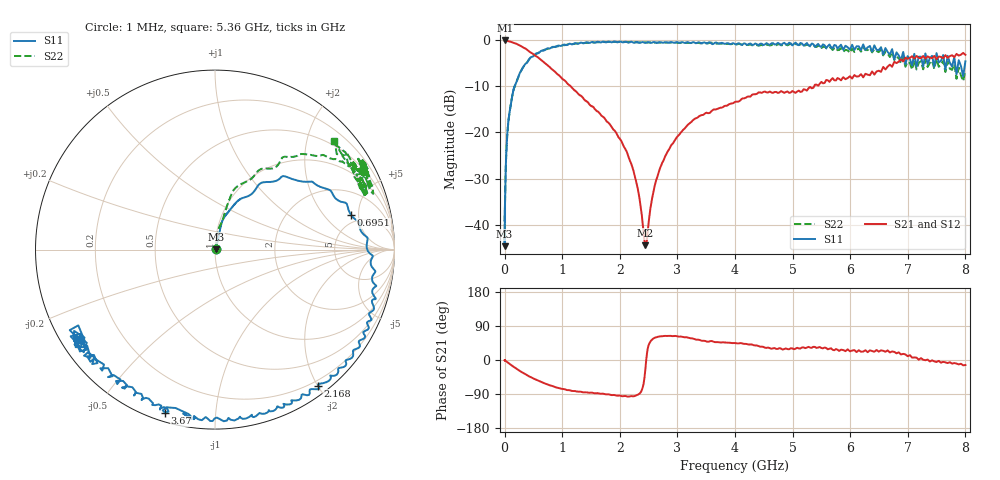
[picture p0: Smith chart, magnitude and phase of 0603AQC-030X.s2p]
!s-Parameter Generated by FASTRON Sdn. Bhd.
!FASTRON P/N : 0603AQC-030X
!Keysight Technologies: E5071C_MY46733604_B.14.02
!Date: Thu Jun 25 13:53:08 2026
!Version  :Rev00  Thu Jun 25 13:53:08 2026
!Data & Calibration Information:
!Freq  S11:SOLT2(ON)  S21:SOLT2(ON)  S12:SOLT2(ON)  S22:SOLT2(ON)
!PortZ  Port1:50+j0  Port2:50+j0
!When reading reference impedance value at option line is always used.
! Remarks : This data is being provided solely for informational purposes.
# Hz S dB R 50
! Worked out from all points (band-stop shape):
!   1601 points, 1 MHz to 8 GHz, reference 50 ohm
!   highest |S21| = -0.01 dB at 6.268 MHz (marker M1); lowest = -44.5 dB at 2.443 GHz (marker M2)
!   |S21| within 3 dB of the highest: start of sweep to 501.9 MHz; 7.84137 GHz to 7.854235 GHz (12.87 MHz wide, 0.164 % of centre)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
!   lowest |S11| = -44.7 dB at 1.297 MHz (marker M3), VSWR 1.01, Z = 50.6 + j0.175 ohm
!   |S11| at or under -10 dB: start of sweep to 171.8 MHz
!   |S22| runs from -43.8 to -0.3 dB; largest |S21 - S12| = 0.012
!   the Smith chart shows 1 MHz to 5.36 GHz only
!   S11 on the Smith chart (normalised r, x): 1 MHz: 1.01, +0.00; 695.1 MHz: 4.05, +4.04; 2.168 GHz: 0.13, -2.01; 3.67 GHz: 0.04, -0.74; 5.36 GHz: 0.05, -0.30
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1000000  -43.10 9.4  -0.07 -0.2  -0.07 -0.1  -41.90 12.2
1297036  -44.70 17.3  -0.07 -0.2  -0.07 -0.1  -42.60 10.2
4479405  -39.00 51.9  -0.07 -0.6  -0.07 -0.6  -39.20 55.7
6268472  -36.70 52.9  -0.01 -0.5  -0.11 -0.3  -37.30 58.8
2.00676e7  -28.30 71.7  -0.09 -2.5  -0.09 -2.5  -28.10 78.3
8.994653e7  -15.40 75.4  -0.24 -10.6  -0.25 -10.5  -15.40 75.8
2.089357e8  -8.97 57.7  -0.75 -23.1  -0.75 -23.1  -8.96 72.0
4.006501e8  -4.65 42.0  -2.09 -41.4  -2.09 -41.4  -4.55 53.4
6.950598e8  -2.13 14.3  -4.86 -61.7  -4.86 -61.8  -2.01 41.5
1.165105e9  -0.85 -13.9  -10.20 -81.5  -10.20 -81.6  -0.81 28.6
1.7949e9  -0.29 -37.2  -17.80 -90.5  -17.90 -90.7  -0.32 30.5
2.167736e9  -0.43 -52.8  -25.80 -96.2  -25.90 -96.3  -0.36 27.4
2.44288e9  -0.53 -63.1  -44.50 -27.0  -44.80 -27.1  -0.46 26.1
2.89772e9  -0.37 -77.0  -22.70 63.3  -22.80 63.4  -0.49 32.4
3.669656e9  -0.44 -107.0  -15.00 47.0  -15.00 46.9  -0.68 26.0
4.115571e9  -0.97 -121.0  -12.70 44.2  -12.70 43.9  -0.91 32.8
4.744521e9  -0.55 -141.0  -11.40 29.4  -11.40 29.1  -0.86 20.4
5.360342e9  -0.82 -147.0  -10.30 34.8  -10.30 34.5  -0.96 42.4
6.110812e9  -1.28 -174.0  -7.85 21.0  -7.83 20.6  -2.04 31.1
6.72769e9  -1.90 -176.0  -5.72 22.5  -5.70 21.9  -2.58 54.9
7.383122e9  -3.84 143.0  -3.74 -4.0  -3.76 -4.8  -4.89 33.1
8e9  -4.54 140.0  -3.13 -13.3  -3.16 -14.0  -6.55 46.2
